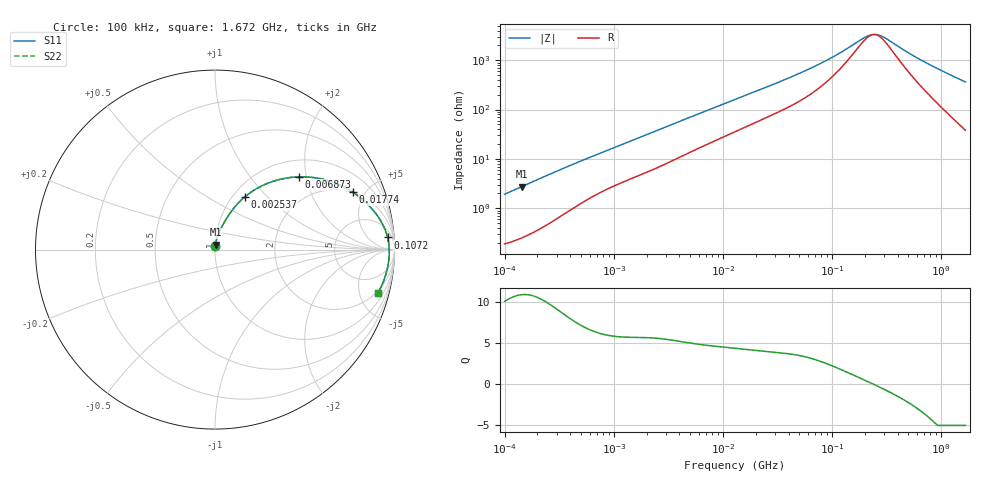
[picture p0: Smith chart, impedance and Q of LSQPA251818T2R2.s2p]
! LSQPA251818T2R2  S-PARAMETER MODEL  ( General Type )
! Model Generated by TAIYO YUDEN Corporation (http://www.ty-top.com)
! Version 3.0
! TAIYO YUDEN Control No. 160907NF25SB-FKC
! Copyright(c) 2007 TAIYO YUDEN CO.,LTD. All Rights Reserved.
! Product Description (link to TY-COMPAS)
! https://ds.yuden.co.jp/TYCOMPAS/or/detail?pn=LSQPA251818T2R2M&u=M
! Products Name : Inductors
! Characteristics :
!  Inductance : 2.2 uH , SRF(min) : 68 MHz , DC Resistance(max) : 0.169 Ohm
!  Rated Current : Saturation :890 mA , Temp Rise : 1100 mA (40 degC)
!  Case Size : 2.5 x 1.8 / 0.098 x 0.071 [mm/inch] , Thickness : 1.8 / 0.071 [mm/inch]
!  (Conditions: Temperature = 25 degC , DC Bias Current/Voltage = 0A / 0V)
! External Node Assignments :
!  1  o---GGG---o  2
! GND o---------o GND
! Frequency Range : 0.1MHz  -  1672.468556MHz  [ 402 STEP ]
# MHz S RI R 50
! Freq[MHz].  S11 Real  S11 Imag  S21 Real  S21 Imag  S12 Real  S12 Imag  S22 Real  S22 Imag
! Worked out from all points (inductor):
!   401 points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, 100 kHz to 1.672 GHz, reference 50 ohm
!   read as one part in series: L = 3.04 uH near 105 kHz
!   highest Q = 10.9 at 144 kHz (marker M1), where L = 3.04 uH
!   self-resonance near 242.7 MHz
!   S11 on the Smith chart (normalised r, x): 100 kHz: 1.00, +0.04; 2.537 MHz: 1.13, +0.75; 6.873 MHz: 1.38, +1.81; 17.74 MHz: 1.97, +4.10; 107.2 MHz: 12, +22; 1.672 GHz: 1.76, -7.21
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0.1  0.00225 0.0191  0.9977 -0.0191  0.9977 -0.0191  0.00225 0.0191
0.144004  0.00326 0.0273  0.9967 -0.0273  0.9967 -0.0273  0.00326 0.0273
0.509815  0.0206 0.0885  0.9794 -0.0885  0.9794 -0.0885  0.0206 0.0885
1.3158  0.0732 0.1877  0.9268 -0.1877  0.9268 -0.1877  0.0732 0.1877
2.536685  0.1668 0.2943  0.8332 -0.2943  0.8332 -0.2943  0.1668 0.2943
2.599112  0.1719 0.2985  0.8281 -0.2985  0.8281 -0.2985  0.1719 0.2985
4.437206  0.3163 0.3781  0.6837 -0.3781  0.6837 -0.3781  0.3163 0.3781
6.873227  0.4677 0.4054  0.5323 -0.4054  0.5323 -0.4054  0.4677 0.4054
12.9324  0.6832 0.3655  0.3168 -0.3655  0.3168 -0.3655  0.6832 0.3655
17.73937  0.7684 0.3196  0.2316 -0.3196  0.2316 -0.3196  0.7684 0.3196
32.57602  0.8795 0.2212  0.1205 -0.2212  0.1205 -0.2212  0.8795 0.2212
65.93127  0.9436 0.1211  0.0564 -0.1211  0.0564 -0.1211  0.9436 0.1211
107.2159  0.9618 0.0679  0.0382 -0.0679  0.0382 -0.0679  0.9618 0.0679
192.159  0.9699 0.0179  0.0301 -0.0179  0.0301 -0.0179  0.9699 0.0179
222.3367  0.9706 0.00669  0.0294 -0.00669  0.0294 -0.00669  0.9706 0.00669
245.0444  0.9709 -0.000735  0.0291 0.000735  0.0291 0.000735  0.9709 -0.000735
270.0712  0.971 -0.00819  0.029 0.00819  0.029 0.00819  0.971 -0.00819
336.1274  0.9707 -0.0254  0.0293 0.0254  0.0293 0.0254  0.9707 -0.0254
484.0384  0.9683 -0.057  0.0317 0.057  0.0317 0.057  0.9683 -0.057
680.2951  0.9628 -0.093  0.0372 0.093  0.0372 0.093  0.9628 -0.093
1106.28  0.9441 -0.1618  0.0559 0.1618  0.0559 0.1618  0.9441 -0.1618
1672.469  0.9074 -0.2418  0.0926 0.2418  0.0926 0.2418  0.9074 -0.2418
